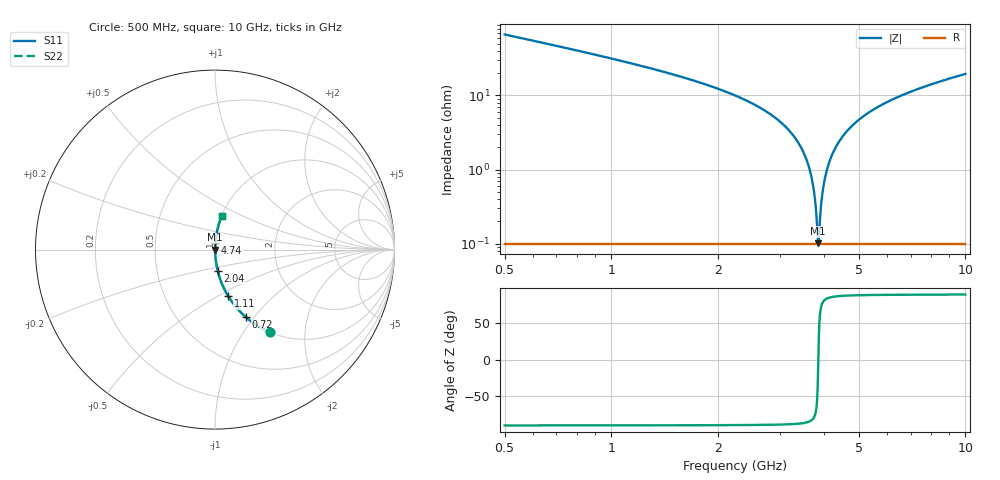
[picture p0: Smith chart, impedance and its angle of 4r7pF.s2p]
! Created Fri Jan 10 15:57:01 2014
# hz S db R 50
! 2 Port Network Data from SP1.SP block
! freq  dbS11  angS11  dbS21  angS21  dbS12  angS12  dbS22  angS22
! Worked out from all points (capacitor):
!   951 points, 500 MHz to 10 GHz, reference 50 ohm
!   read as one part in series: C = 4.7 pF near 540 MHz
!   lowest |Z| = 100 mohm at 3.84 GHz (marker M1)
!   series resonance near 3.844 GHz, so ESL is about 360 pH
!   S11 on the Smith chart (normalised r, x): 500 MHz: 1.00, -1.33; 720 MHz: 1.00, -0.91; 1.11 GHz: 1.00, -0.56; 2.04 GHz: 1.00, -0.24; 4.74 GHz: 1.00, +0.07; 10 GHz: 1.00, +0.39
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5e8  -5.13 -56.3  -1.60 33.6  -1.60 33.6  -5.13 -56.3
7.2e8  -7.68 -65.5  -0.82 24.4  -0.82 24.4  -7.68 -65.5
1.11e9  -11.40 -74.2  -0.33 15.6  -0.33 15.6  -11.40 -74.2
2.04e9  -18.54 -82.7  -0.07 6.8  -0.07 6.8  -18.54 -82.7
2.09e9  -18.92 -83.0  -0.06 6.5  -0.06 6.5  -18.92 -83.0
2.74e9  -24.35 -85.6  -0.02 3.5  -0.02 3.5  -24.35 -85.6
3.18e9  -29.48 -86.4  -0.01 1.9  -0.01 1.9  -29.48 -86.4
3.48e9  -35.11 -85.8  -0.01 1.0  -0.01 1.0  -35.11 -85.8
3.67e9  -41.72 -82.6  -0.01 0.5  -0.01 0.5  -41.72 -82.6
3.74e9  -46.17 -78.1  -0.01 0.3  -0.01 0.3  -46.17 -78.1
3.81e9  -54.72 -57.3  -0.01 0.1  -0.01 0.1  -54.72 -57.3
3.84e9  -59.97 -9.6  -0.01 0.0  -0.01 0.0  -59.97 -9.6
3.87e9  -56.15 50.5  -0.01 -0.1  -0.01 -0.1  -56.15 50.5
3.92e9  -48.87 73.9  -0.01 -0.2  -0.01 -0.2  -48.87 73.9
3.97e9  -44.76 79.8  -0.01 -0.3  -0.01 -0.3  -44.76 79.8
4.11e9  -38.53 84.5  -0.01 -0.7  -0.01 -0.7  -38.53 84.5
4.36e9  -33.05 86.2  -0.01 -1.3  -0.01 -1.3  -33.05 86.2
4.74e9  -28.60 86.3  -0.01 -2.1  -0.01 -2.1  -28.60 86.3
5.25e9  -25.08 85.8  -0.02 -3.2  -0.02 -3.2  -25.08 85.8
6.84e9  -19.45 83.4  -0.06 -6.1  -0.06 -6.1  -19.45 83.4
8.42e9  -16.43 81.0  -0.11 -8.7  -0.11 -8.7  -16.43 81.0
1e10  -14.35 78.7  -0.17 -11.0  -0.17 -11.0  -14.35 78.7
